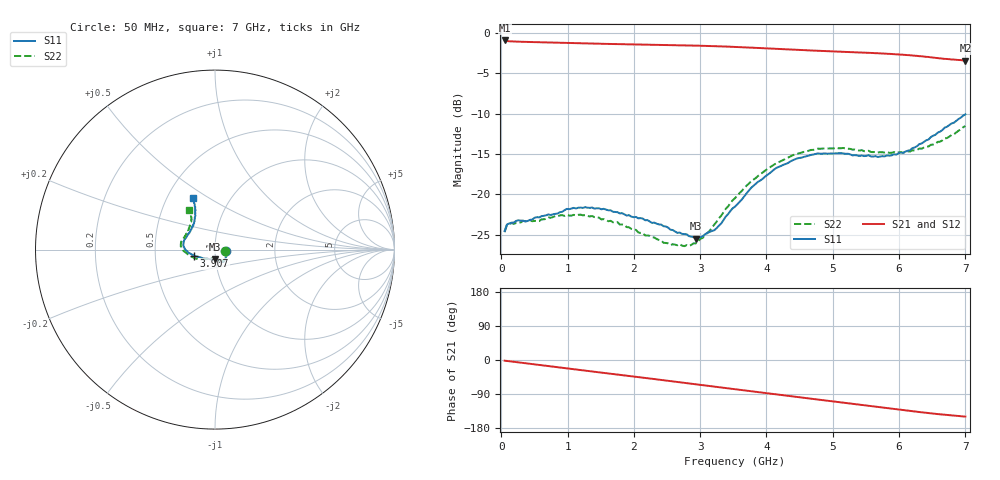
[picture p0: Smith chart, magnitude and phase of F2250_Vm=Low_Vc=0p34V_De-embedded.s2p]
! Integrated Device Technology
! Corporate Headquarters
! 6024 Silver Creek Valley Road
! San Jose, CA 95138  USA
! Phone:  1-408-284-8200
! Toll Free:  1-800-223-1366
! Webpage:  http://www.idt.com/
! Timing and RF Division
! 515 Groton Road, Suite 102
! Westford, MA 01886-6024
! Device:  F2250
! Description: Voltage Variable RF Attenuator
! Frequency:  50.0 -  6000.00 MHz
! Package:  3x3 mm Thin QFN Plastic Package: 16 pin
! Ports:  2 RF, 3 DC
!  Pin  1  = GND
!  Pin  2  = NC
!  Pin  3  = RF1  = Port 1
!  Pin  4  = NC
!  Pin  5  = GND
!  Pin  6  = GND
!  Pin  7  = GND
!  Pin  8  = GND
!  Pin  9  = NC
!  Pin 10  = RF2  = Port 2
!  Pin 11  = NC
!  Pin 12  = GND
!  Pin 13  = GND
!  Pin 14  = VCNTRL
!  Pin 15  = VDD
!  Pin 16  = VMODE
! Vcntrl:  0.340 Volts
! Vmode:  +0.000 Volts
! Vdd:  +3.30  Volts
! Current:  1.117 mA
! Data:  The device was measured on a the F2250 evaluation board which has
!  individual transmission lines to the RF pins.  Data was collected
!  using a calibrated network analyzer.  The evaluation board was
!  de-embedded using a TRL calibration technique.
!  The reference plane is the edge of the package pin.
! Misc:  SN 10
!  Action Tracker AT0258
! Date Measured:  2014-11-26
! Date:  2015-10-15  MJV
! Note:
!  Integrated Device Technology supplies this data as a sample of measured
!  data at the package pin for this product.  Your particular data for this
!  product may vary.
!  Data was taken at 25 degrees C.
!  Integrated Device Technology reserves the right to change this data at anytime.
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# GHz S dB R 50
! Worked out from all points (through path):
!   201 points, 50 MHz to 7 GHz, reference 50 ohm
!   highest |S21| = -0.96 dB at 50 MHz (marker M1); lowest = -3.4 dB at 7 GHz (marker M2)
!   group delay of S21, straight-line fit = 60 ps
!   lowest |S11| = -25.5 dB at 2.934 GHz (marker M3), VSWR 1.11, Z = 49.8 - j5.33 ohm
!   |S11| at or under -10 dB: start of sweep to end of sweep
!   |S22| runs from -26.4 to -11.5 dB; largest |S21 - S12| = 0.00036
!   S11 on the Smith chart (normalised r, x): 50 MHz: 1.12, -0.02; 3.907 GHz: 0.79, -0.05; 7 GHz: 0.67, +0.43
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0.05  -24.52 -9.1  -0.96 -1.8  -0.96 -1.8  -24.66 -9.6
0.08475  -23.71 -9.1  -1.04 -2.5  -1.03 -2.5  -23.79 -9.0
0.15425  -23.49 -11.3  -1.08 -4.0  -1.08 -4.0  -23.55 -10.7
0.57125  -22.84 -28.8  -1.18 -13.1  -1.18 -13.1  -23.29 -29.7
0.71025  -22.48 -36.8  -1.21 -16.2  -1.21 -16.2  -22.84 -37.7
1.2315  -21.66 -54.2  -1.32 -27.4  -1.32 -27.4  -22.59 -58.6
1.75275  -22.19 -60.9  -1.42 -38.4  -1.41 -38.4  -23.42 -66.1
2.37825  -23.70 -61.9  -1.51 -51.8  -1.50 -51.8  -25.63 -68.6
2.552  -24.36 -65.9  -1.53 -55.6  -1.53 -55.6  -26.26 -74.3
2.83  -25.15 -80.5  -1.58 -61.7  -1.58 -61.7  -26.38 -92.9
2.93425  -25.45 -89.1  -1.60 -64.0  -1.60 -64.0  -26.05 -101.4
3.21225  -24.42 -118.3  -1.67 -70.2  -1.67 -70.2  -23.73 -126.6
3.525  -21.50 -145.5  -1.76 -77.1  -1.76 -77.1  -20.46 -145.6
3.76825  -19.18 -159.3  -1.85 -82.5  -1.85 -82.5  -18.37 -156.1
3.90725  -18.27 -163.8  -1.91 -85.5  -1.90 -85.5  -17.50 -162.2
4.1505  -16.71 -172.2  -2.01 -90.8  -2.00 -90.8  -16.15 -170.9
4.7065  -15.06 173.3  -2.22 -102.9  -2.22 -102.9  -14.49 175.9
5.15825  -14.93 162.6  -2.37 -112.6  -2.37 -112.6  -14.25 166.7
5.85325  -15.22 139.4  -2.62 -127.5  -2.62 -127.6  -14.87 151.6
6.166  -14.53 128.3  -2.79 -134.4  -2.79 -134.4  -14.69 142.7
6.444  -13.21 119.9  -3.00 -140.1  -3.00 -140.2  -14.08 133.3
7  -10.10 113.4  -3.44 -149.4  -3.45 -149.4  -11.54 123.9
